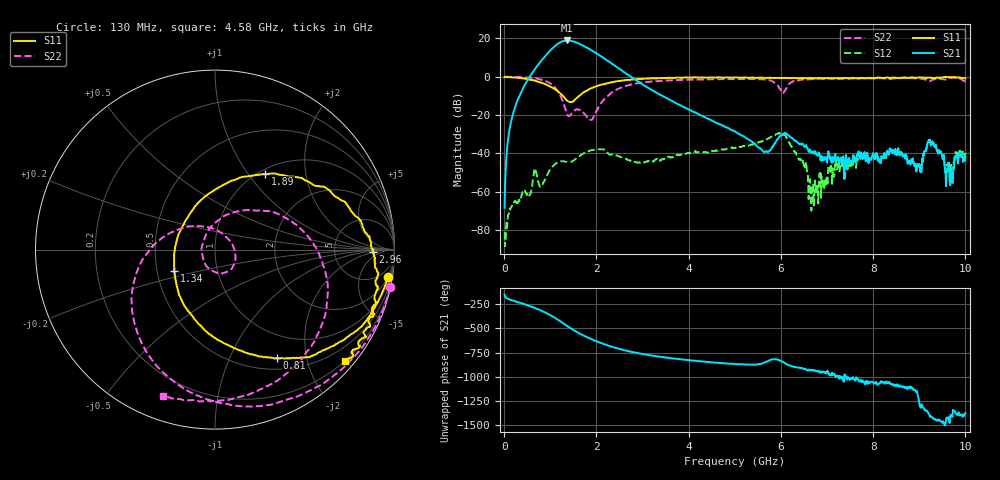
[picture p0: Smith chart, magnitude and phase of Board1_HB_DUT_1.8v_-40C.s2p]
! Created Tue May 27 11:34:49 2025
# hz S ma R 50
! 2 Port Network Data from SP1.SP block
! freq  magS11  angS11  magS21  angS21  magS12  angS12  magS22  angS22
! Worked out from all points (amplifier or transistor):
!   1000 points, 10 MHz to 10 GHz, reference 50 ohm
!   highest |S21| = 19.0 dB at 1.36 GHz (marker M1)
!   |S21| within 3 dB of that: 1.096 GHz to 1.736 GHz (639.7 MHz wide, 45.2 % of centre)
!   unconditionally stable (mu >= 1): 19.91 MHz to 20.99 MHz; 86.75 MHz to 109.6 MHz; 110.4 MHz to end of sweep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
!   at 1.67 GHz: K = 6.85, MAG = 17.4 dB, |S12| = -40.7 dB
!   at 5.01 GHz: K = 11.54, MAG = -9.4 dB, |S12| = -37.0 dB
!   at 10 GHz: K = 390.96, MAG = -30.0 dB, |S12| = -39.6 dB
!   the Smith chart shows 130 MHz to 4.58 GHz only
!   S11 on the Smith chart (normalised r, x): 130 MHz: 2, -12; 810 MHz: 0.65, -1.52; 1.34 GHz: 0.61, -0.16; 1.89 GHz: 1.07, +1.21; 2.96 GHz: 15, -2; 4.58 GHz: 0.20, -2.69
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1e7  0.9815 -1.0  0.0003832 -152.7  8.904e-05 87.6  1.005 -0.8
1.3e8  0.9747 -9.1  0.05166 155.1  0.0003431 78.5  0.9985 -11.9
5.6e8  0.8461 -39.5  1.039 88.6  0.0008632 114.0  0.9476 -55.9
8.1e8  0.6951 -60.2  2.678 40.2  0.00139 98.5  0.8449 -90.5
9.6e8  0.59 -74.5  4.33 5.7  0.003218 119.2  0.719 -117.7
1.11e9  0.4697 -94.3  6.509 -35.5  0.005359 100.5  0.5154 -153.5
1.24e9  0.348 -120.5  8.22 -76.2  0.006269 82.4  0.2824 163.3
1.34e9  0.257 -152.2  8.854 -109.0  0.006098 73.5  0.1295 106.6
1.36e9  0.242 -160.5  8.883 -115.4  0.006067 73.5  0.112 89.4
1.51e9  0.2351 130.4  8.308 -161.0  0.006626 77.1  0.1272 -27.5
1.68e9  0.3576 83.8  6.808 154.5  0.009366 71.1  0.1268 -87.5
1.89e9  0.5062 56.4  4.954 107.8  0.01213 48.9  0.07529 162.6
2.22e9  0.6722 31.8  2.741 47.2  0.01149 4.3  0.2974 47.5
2.54e9  0.7919 15.3  1.498 1.5  0.007979 -0.8  0.5266 7.6
2.96e9  0.8785 -1.0  0.6797 -41.9  0.005901 9.7  0.7007 -27.5
3.34e9  0.92 -12.5  0.3632 -70.9  0.006395 13.2  0.7764 -51.0
4.58e9  0.9519 -40.5  0.06459 -134.5  0.01161 1.6  0.8645 -109.6
5.01e9  0.9719 -48.1  0.03718 -148.9  0.01407 -8.4  0.8755 -126.4
6.05e9  0.9318 -69.2  0.03247 -126.7  0.03252 -102.8  0.3753 -152.0
6.67e9  0.923 -87.4  0.01032 150.7  0.0009581 -128.6  0.8778 -156.3
8.34e9  0.9398 -134.1  0.009271 14.7  0.00911 8.8  0.8683 164.2
1e10  0.9098 -164.1  0.008265 65.2  0.01052 62.5  0.7786 128.4
